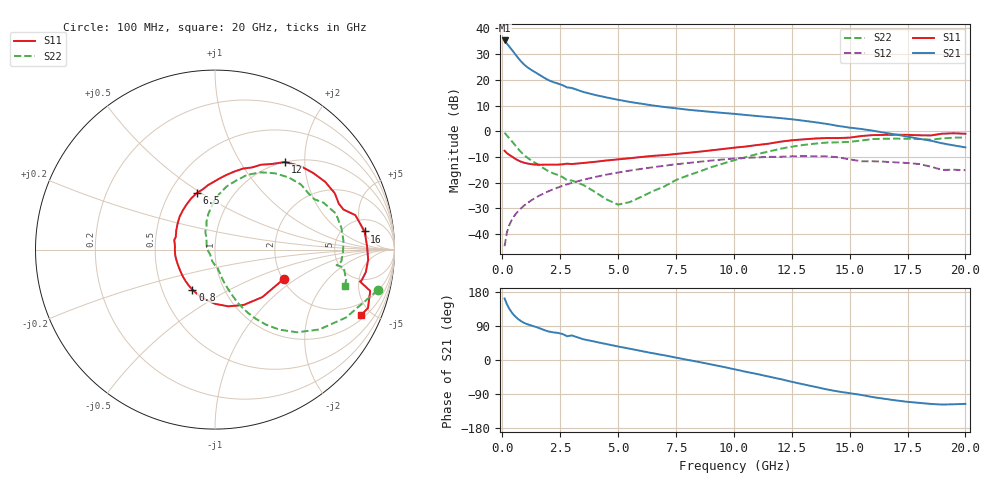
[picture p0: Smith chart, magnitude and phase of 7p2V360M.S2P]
! Infineon Technologies  Discrete & RF Semiconductors
! bfp620
! VCE =  2.3 V,  IC =  60 mA
! Common Emitter S-Parameters:  Sep 2002
# GHz  S  MA  R  50
!  f  S11  S21  S12  S22
! GHz  MAG  ANG  MAG  ANG  MAG  ANG  MAG  ANG
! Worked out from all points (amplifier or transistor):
!   59 points, 100 MHz to 20 GHz, reference 50 ohm
!   highest |S21| = 35.3 dB at 100 MHz (marker M1)
!   |S21| within 3 dB of that: start of sweep to 356 MHz
!   unconditionally stable (mu >= 1): 2.542 GHz to 9.82 GHz; 17.2 GHz to end of sweep
!   at 1 GHz: K = 0.87, MSG = 27.0 dB, |S12| = -28.5 dB
!   at 5.5 GHz: K = 1.04, MAG = 12.2 dB, |S12| = -15.3 dB
!   at 20 GHz: K = 1.24, MAG = 1.5 dB, |S12| = -15.2 dB
!   S11 on the Smith chart (normalised r, x): 100 MHz: 2.03, -0.80; 800 MHz: 0.71, -0.34; 6.5 GHz: 0.68, +0.48; 12 GHz: 1.00, +1.60; 16 GHz: 7.79, +5.33; 20 GHz: 1.21, -4.34
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0.1  0.4168 -23.1  58.31 162.5  0.0058 72.3  0.9354 -13.9
0.2  0.3737 -45.1  50.41 147.3  0.0107 71.2  0.8224 -27.4
0.3  0.3474 -62.6  44.37 135.5  0.0148 69.8  0.7315 -37.5
0.4  0.3243 -77.0  39.01 126.2  0.0185 68.7  0.6489 -45.2
0.5  0.3027 -89.5  34.13 118.7  0.0219 67.8  0.5725 -51.2
0.6  0.2837 -100.7  29.81 112.5  0.0252 67.1  0.5041 -55.9
0.7  0.2683 -110.6  26.13 107.2  0.0283 66.5  0.4453 -59.6
0.8  0.2562 -119.3  23.11 102.9  0.0313 66.1  0.3966 -62.5
0.9  0.2471 -126.8  20.71 99.3  0.0344 65.8  0.3573 -64.7
1.1  0.2346 -138.7  17.35 94.0  0.0404 65.1  0.3009 -67.8
1.9  0.2235 -171.0  10.38 77.1  0.065 60.6  0.1764 -75.3
2.8  0.2337 166.6  7.121 62.6  0.0926 53.5  0.1114 -81.5
3.5  0.2412 153.4  5.805 54.7  0.1137 47.2  0.0899 -88.7
5  0.2833 129.0  4.089 35.6  0.1572 33.1  0.0373 -140.2
6.5  0.3311 107.9  3.169 17.8  0.1987 18.8  0.0681 133.7
7  0.3427 101.4  2.958 12.4  0.2129 14.0  0.0843 124.7
10.5  0.5023 65.7  2.072 -30.8  0.3023 -25.2  0.3121 85.3
12  0.6243 51.4  1.801 -50.2  0.3178 -42.8  0.4544 66.6
13.5  0.7208 31.6  1.498 -70.7  0.3256 -61.8  0.5736 44.7
16  0.8397 6.9  1.024 -97.9  0.2608 -85.9  0.7027 16.6
17  0.8553 -3.8  0.862 -106.6  0.2478 -93.9  0.717 4.1
20  0.8924 -24.2  0.485 -115.8  0.1742 -103.2  0.7529 -15.8
